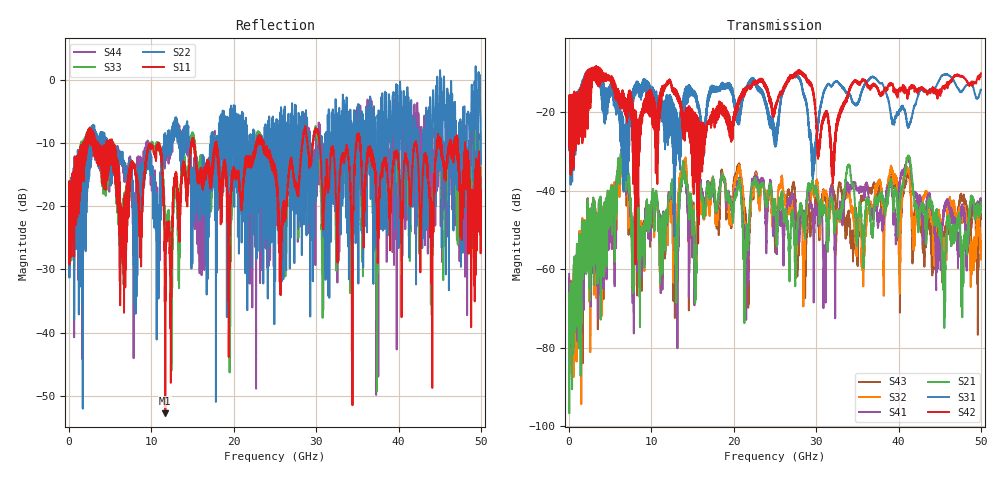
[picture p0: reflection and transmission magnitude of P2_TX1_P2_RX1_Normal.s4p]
!Keysight Technologies,N5225B,MY57041031,A.13.20.10
!Date: Friday, May 31, 2019 11:27:17
!Correction: S11(Full 4 Port(1,2,3,4))
!S12(Full 4 Port(1,2,3,4))
!S13(Full 4 Port(1,2,3,4))
!S14(Full 4 Port(1,2,3,4))
!S21(Full 4 Port(1,2,3,4))
!S22(Full 4 Port(1,2,3,4))
!S23(Full 4 Port(1,2,3,4))
!S24(Full 4 Port(1,2,3,4))
!S31(Full 4 Port(1,2,3,4))
!S32(Full 4 Port(1,2,3,4))
!S33(Full 4 Port(1,2,3,4))
!S34(Full 4 Port(1,2,3,4))
!S41(Full 4 Port(1,2,3,4))
!S42(Full 4 Port(1,2,3,4))
!S43(Full 4 Port(1,2,3,4))
!S44(Full 4 Port(1,2,3,4))
!S4P File: Measurements: <S11,S12,S13,S14>,
!<S21,S22,S23,S24>,
!<S31,S32,S33,S34>,
!<S41,S42,S43,S44>:
# Hz S  dB  R 50.0
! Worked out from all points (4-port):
!   5000 points, 10 MHz to 50 GHz, reference 50 ohm
!   strongest paths, dB at 10 MHz, 12.51 GHz, 25.01 GHz, 37.51 GHz, 50 GHz:
!     S42: -19.4, -14.0, -19.7, -14.1, -10.1
!     S31: -19.4, -17.3, -28.8, -12.1, -14.3
!     S21: -67.0, -37.1, -42.8, -43.2, -42.8
!     S41: -61.2, -38.9, -46.3, -49.5, -42.7
!     S32: -70.0, -41.1, -48.4, -38.2, -57.5
!     S43: -62.2, -41.9, -52.3, -40.8, -45.9
!   lowest |S11| = -52.8 dB at 11.69 GHz (marker M1), VSWR 1.00, Z = 49.8 - j0.138 ohm
!   |S11| at or under -10 dB: 5.36 GHz to 10.81 GHz (5.449 GHz wide, 67.4 % of centre); 17.89 GHz to 22.7 GHz (4.804 GHz wide, 23.7 % of centre); 35.31 GHz to 41.98 GHz (6.665 GHz wide, 17.2 % of centre)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
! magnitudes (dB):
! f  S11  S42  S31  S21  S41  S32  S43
! 10 MHz  -19.6  -19.4  -19.4  -67.0  -61.2  -70.0  -62.2
! 6.56 GHz  -20.3  -16.1  -22.5  -33.1  -32.2  -32.9  -32.1
! 11.69 GHz  -52.8  -13.4  -23.0  -52.1  -51.6  -50.0  -49.7
! 28.01 GHz  -14.2  -9.9  -11.6  -45.3  -49.9  -49.1  -46.4
! 29.65 GHz  -9.5  -14.6  -35.9  -38.7  -51.0  -40.3  -47.6
! 32.02 GHz  -11.2  -33.6  -13.0  -42.9  -41.3  -44.3  -39.5
! 50 GHz  -17.6  -10.1  -14.3  -42.8  -42.7  -57.5  -45.9
